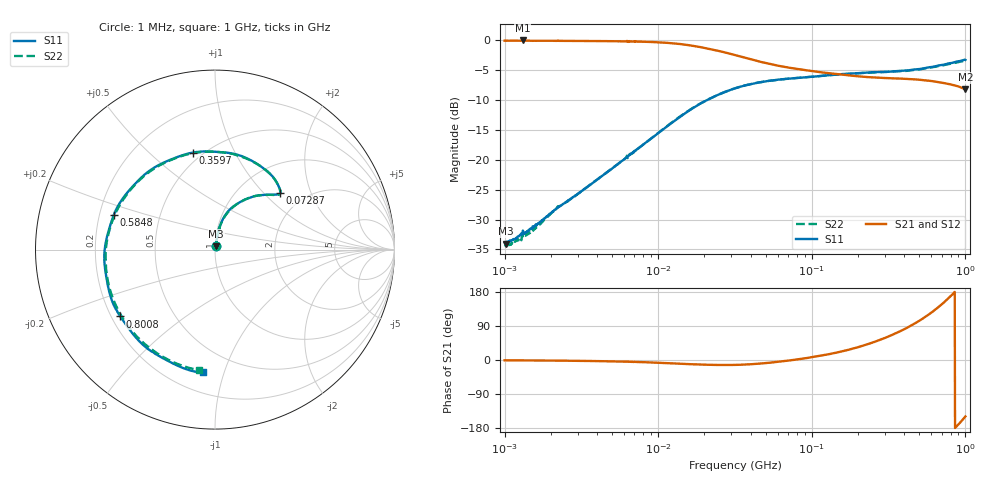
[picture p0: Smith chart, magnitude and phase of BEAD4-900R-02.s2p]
!s-Parameter Generated by FASTRON Sdn. Bhd.
!FASTRON P/N : BEAD/4-900R
!Vector Network Analyser E5071C,MY46733604,B.14.02
!Date: Mon Jul 31 13:14:17 2023
!Data & Calibration Information:
!Freq	S11:SOLT2(ON)	S21:SOLT2(ON)	S12:SOLT2(ON)	S22:SOLT2(ON)
!PortZ  Port1:50+j0  Port2:50+j0
!When reading, reference impedance value at option line is always used.
! Remarks : This data is being provided solely for informational purposes.
# Hz S dB R 50
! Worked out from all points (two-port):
!   1601 points, 1 MHz to 1 GHz, reference 50 ohm
!   highest |S21| = 0.00 dB at 1.316 MHz (marker M1); lowest = -8.2 dB at 1 GHz (marker M2)
!   |S21| within 3 dB of the highest: start of sweep to 37.99 MHz
!   lowest |S11| = -34.1 dB at 1.025 MHz (marker M3), VSWR 1.04, Z = 50.6 + j1.9 ohm
!   |S11| at or under -10 dB: start of sweep to 20.75 MHz
!   |S22| runs from -34.5 to -3.4 dB; largest |S21 - S12| = 0.0048
!   S11 on the Smith chart (normalised r, x): 1 MHz: 1.01, +0.04; 72.87 MHz: 1.52, +1.25; 359.7 MHz: 0.45, +0.70; 584.8 MHz: 0.26, +0.16; 800.8 MHz: 0.24, -0.30; 1 GHz: 0.33, -0.85
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1000000  -33.90 70.0  -0.04 -0.8  -0.05 -0.8  -34.14 69.7
1025491  -34.05 70.8  -0.05 -0.9  -0.05 -0.9  -34.46 71.6
1316094  -31.84 75.5  -0.00 -1.0  -0.01 -1.0  -32.54 71.9
3167252  -25.23 80.3  -0.09 -2.4  -0.09 -2.3  -25.26 79.9
1.002882e7  -15.51 76.0  -0.31 -7.2  -0.32 -7.2  -15.47 75.6
1.796978e7  -10.88 63.9  -1.03 -11.8  -1.03 -11.7  -10.84 63.6
3.163788e7  -8.02 49.9  -2.45 -12.9  -2.45 -12.9  -8.01 49.8
4.829672e7  -6.91 42.7  -3.69 -8.7  -3.68 -8.7  -6.92 42.4
7.2867e7  -6.37 40.9  -4.61 -0.7  -4.60 -0.7  -6.37 40.7
1.00144e8  -6.08 43.7  -5.12 7.3  -5.12 7.4  -6.08 43.6
1.46044e8  -5.70 52.0  -5.65 19.8  -5.65 19.8  -5.72 51.7
1.988072e8  -5.49 63.2  -6.00 33.5  -6.00 33.6  -5.50 63.0
2.531682e8  -5.31 76.1  -6.20 47.2  -6.19 47.2  -5.37 75.5
3.171813e8  -5.25 91.7  -6.33 62.4  -6.32 62.4  -5.26 91.2
3.597203e8  -5.12 102.7  -6.37 72.3  -6.36 72.3  -5.18 102.0
4.634253e8  -4.87 129.5  -6.51 95.4  -6.51 95.4  -4.95 128.8
5.343269e8  -4.68 147.6  -6.66 110.8  -6.65 110.8  -4.75 147.1
5.847993e8  -4.50 161.0  -6.76 121.7  -6.75 121.8  -4.58 160.1
6.884005e8  -4.15 -172.8  -7.03 144.1  -7.03 144.2  -4.25 -173.7
8.008438e8  -3.80 -144.8  -7.36 168.3  -7.37 168.4  -3.90 -145.8
9.004219e8  -3.49 -120.2  -7.70 -170.3  -7.72 -170.2  -3.62 -121.4
1e9  -3.26 -95.7  -8.20 -149.0  -8.19 -148.8  -3.39 -97.4
